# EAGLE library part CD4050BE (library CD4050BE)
CD4050BE, Hex Inverter Buffer, Converter, 26mA -0.5 20 V 16-Pin PDIP Source: Datasheet
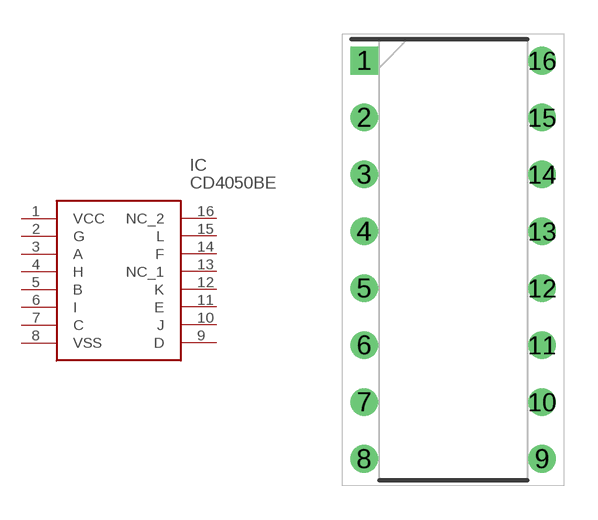
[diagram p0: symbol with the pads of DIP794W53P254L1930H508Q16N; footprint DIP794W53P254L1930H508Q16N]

Designator prefix IC

## CD4050BE (Arrow_Part_Number: CD4050BE; Arrow_Price-Stock: https://www.arrow.com/en/products/cd4050be/texas-instruments?utm_currency=USD&region=nac; Description: CD4050BE, Hex Inverter Buffer, Converter, 26mA -0.5 20 V 16-Pin PDIP; Height: 5.08mm; Manufacturer_Name: Texas Instruments; Manufacturer_Part_Number: CD4050BE; Mouser_Part_Number: 595-CD4050BE; Mouser_Price-Stock: https://www.mouser.co.uk/ProductDetail/Texas-Instruments/CD4050BE?qs=j%2FZo4ajzVJLKLpJvKsajlg%3D%3D)  [DIP794W53P254L1930H508Q16N]
1  VCC
2  G
3  A
4  H
5  B
6  I
7  C
8  VSS
9  D
10  J
11  E
12  K
13  NC_1
14  F
15  L
16  NC_2

## Footprint DIP794W53P254L1930H508Q16N (pad centres in mm)
N (R-PDIP-T)
drill 0.73 pad 1.13 square: 1 -3.97,8.89
drill 0.73 pad 1.13: 2 -3.97,6.35; 3 -3.97,3.81; 4 -3.97,1.27; 5 -3.97,-1.27; 6 -3.97,-3.81; 7 -3.97,-6.35; 8 -3.97,-8.89; 9 3.97,-8.89; 10 3.97,-6.35; 11 3.97,-3.81; 12 3.97,-1.27; 13 3.97,1.27; 14 3.97,3.81; 15 3.97,6.35; 16 3.97,8.89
